| IBIS file stm32u3b5_3c5_lqfp100_smps.ibs
[IBIS ver] 4.2
[File name] stm32u3b5_3c5_lqfp100_smps.ibs
[File Rev] 0.1
[Date] 09-03-2026
[Source] Data Created at STMicroelectronics
[Notes]  File originated from ELDO simulations.
[Disclaimer]  This information is for modeling purpose only and is
   not guaranted. The information is subject to change without
   notice.
[Copyright] Copyright 2026 STMicroelectronics Inc.
|   Component stm32u3b5_3c5_lqfp100_smps
[Component] stm32u3b5_3c5_lqfp100_smps
[Manufacturer] STMicroelectronics
[Package]
| variable   typ   min   max
R_pkg  0  NA  NA
L_pkg  0  NA  NA
C_pkg  0  NA  NA
[Pin]   signal_name   model_name
1  PE2  io8_ft_100m
2  PE3  io8_ft_100m_hslv
3  PE4  io8_ft_100m
4  PE5  io8_ft_100m
5  PE6  io8_ft_100m
6  VBAT  power
7  PC13  io8_ft_100m_v33
8  PC14-OSC32_IN  io_ft_tamp
9  PC15-OSC32_OUT  io_ft_tamp
10  VSS  gnd
11  VDD  power
12  PH0-OSC_IN  io8_ft_100m
13  PH1-OSC_OUT  io8_ft_100m
14  NRST  ioreset_v33
15  PC0  io8_ft_100m_hslv
16  PC1  io8_ft_100m_hslv
17  PC2  io8_ft_100m_hslv
18  PC3  io8_ft_100m_hslv
19  VSSA_VREFM  nc
20  VREFP  nc
21  VDDA  nc
22  PA0  io8_ft_100m
23  PA1  io8_ft_100m_hslv
24  PA2  io8_ft_100m_hslv
25  PA3  io8_ft_100m_hslv
26  VSS  gnd
27  VDD  power
28  PA4  io8_ft_100m_hslv
29  PA5  io8_ft_100m
30  PA6  io8_ft_100m_hslv
31  PA7  io8_ft_100m_hslv
32  PB0  io8_ft_100m_hslv
33  PB1  io8_ft_100m_hslv
34  PB2  io8_ft_100m_hslv
35  PE7  io8_ft_100m
36  PE8  io8_ft_100m
37  PE9  io8_ft_100m_hslv
38  PE10  io8_ft_100m_hslv
39  PE11  io8_ft_100m_hslv
40  PE12  io8_ft_100m_hslv
41  PE13  io8_ft_100m_hslv
42  PE14  io8_ft_100m_hslv
43  PE15  io8_ft_100m_hslv
44  PB10  io8_ft_100m_hslv
45  PB11  io8_ft_100m_hslv
46  VLXSMPS  nc
47  VDDSMPS  nc
48  VSSSMPS  nc
49  VDD11  nc
50  VSS  gnd
51  VDD  power
52  PB13  io8_ft_100m_hslv
53  PB14  io8_ft_100m_hslv
54  PB15  io8_ft_100m
55  PD8  io8_ft_100m
56  PD9  io8_ft_100m
57  PD10  io8_ft_100m
58  PD11  io8_ft_100m_hslv
59  PD12  io8_ft_100m_hslv
60  PD13  io8_ft_100m_hslv
61  PD14  io8_ft_100m
62  PD15  io8_ft_100m
63  PC6  io8_ft_100m_hslv
64  PC7  io8_ft_100m_hslv
65  PC8  io8_ft_100m_hslv
66  PC9  io8_ft_100m_hslv
67  PA8  io8_ft_100m_hslv
68  PA9  io8_ft_100m
69  PA10  io8_ft_100m
70  PA11  io8usb_ft_phy
71  PA12  io8usb_ft_phy
72  PA13  io8_ft_100m
73  VDDUSB  power
74  VSS  gnd
75  VDD  power
76  PA14  io8_ft_100m
77  PA15  io8_ft_100m
78  PC10  io8_ft_100m_hslv
79  PC11  io8_ft_100m_hslv
80  PC12  io8_ft_100m_hslv
81  PD0  io8_ft_100m
82  PD1  io8_ft_100m
83  PD2  io8_ft_100m_hslv
84  PD3  io8_ft_100m_hslv
85  PD4  io8_ft_100m_hslv
86  PD5  io8_ft_100m_hslv
87  PD6  io8_ft_100m_hslv
88  PD7  io8_ft_100m_hslv
89  PB3  io8_ft_100m_hslv
90  PB4  io8_ft_100m_hslv
91  PB5  io8_ft_100m_hslv
92  PB6  io8_ft_100m_hslv
93  PB7  io8_ft_100m_hslv
94  PH3-BOOT0  io8_ft_100m_hslv
95  PB8  io8_ft_100m_hslv
96  PB9  io8_ft_100m_hslv
97  PE0  io8_ft_100m
98  VDD11  nc
99  VSS  gnd
100  VDD  power
[Package Model]   42a-lqfp-14x14-100-251212
[Pin Mapping]   pulldown_ref   pullup_ref   | Comment
1  gndio  vddio
2  gndio  vddio
3  gndio  vddio
4  gndio  vddio
5  gndio  vddio
6  nc  vsw
7  gndio  vsw
8  gndio  vsw
9  gndio  vsw
10  gndio  nc
11  nc  vddio
12  gndio  vddio
13  gndio  vddio
14  gndio  vddio
15  gndio  vddio
16  gndio  vddio
17  gndio  vddio
18  gndio  vddio
19  nc  nc
20  nc  nc
21  nc  nc
22  gndio  vddio
23  gndio  vddio
24  gndio  vddio
25  gndio  vddio
26  gndio  nc
27  nc  vddio
28  gndio  vddio
29  gndio  vddio
30  gndio  vddio
31  gndio  vddio
32  gndio  vddio
33  gndio  vddio
34  gndio  vddio
35  gndio  vddio
36  gndio  vddio
37  gndio  vddio
38  gndio  vddio
39  gndio  vddio
40  gndio  vddio
41  gndio  vddio
42  gndio  vddio
43  gndio  vddio
44  gndio  vddio
45  gndio  vddio
46  nc  nc
47  nc  nc
48  nc  nc
49  nc  nc
50  gndio  nc
51  nc  vddio
52  gndio  vddio
53  gndio  vddio
54  gndio  vddio
55  gndio  vddio
56  gndio  vddio
57  gndio  vddio
58  gndio  vddio
59  gndio  vddio
60  gndio  vddio
61  gndio  vddio
62  gndio  vddio
63  gndio  vddio
64  gndio  vddio
65  gndio  vddio
66  gndio  vddio
67  gndio  vddio
68  gndio  vddio
69  gndio  vddio
70  gndio  vddusb  | Depending on IO usage
| 70  gndio  vddio  | Depending on IO usage
71  gndio  vddusb  | Depending on IO usage
| 71  gndio  vddio  | Depending on IO usage
72  gndio  vddio
73  nc  vddusb
74  gndio  nc
75  nc  vddio
76  gndio  vddio
77  gndio  vddio
78  gndio  vddio
79  gndio  vddio
80  gndio  vddio
81  gndio  vddio
82  gndio  vddio
83  gndio  vddio
84  gndio  vddio
85  gndio  vddio
86  gndio  vddio
87  gndio  vddio
88  gndio  vddio
89  gndio  vddio
90  gndio  vddio
91  gndio  vddio
92  gndio  vddio
93  gndio  vddio
94  gndio  vddio
95  gndio  vddio
96  gndio  vddio
97  gndio  vddio
98  nc  nc
99  gndio  nc
100  nc  vddio
|[Diff Pin]  inv_pin  vdiff  tdelay_typ  tdelay_min  tdelay_max
|71  70  NA  NA  NA  NA
[Model Selector] io8_ft_100m
io8_ft_100m_ls_1v2  "GPIO 100MHz - 5V tolerant - low speed - 1.2V range"
io8_ft_100m_ls_1v8  "GPIO 100MHz - 5V tolerant - low speed - 1.8V range"
io8_ft_100m_ls_3v3  "GPIO 100MHz - 5V tolerant - low speed - 3.3V range"
io8_ft_100m_ms_1v2  "GPIO 100MHz - 5V tolerant - med speed - 1.2V range"
io8_ft_100m_ms_1v8  "GPIO 100MHz - 5V tolerant - med speed - 1.8V range"
io8_ft_100m_ms_3v3  "GPIO 100MHz - 5V tolerant - med speed - 3.3V range"
io8_ft_100m_fs_1v2  "GPIO 100MHz - 5V tolerant - fast speed - 1.2V range"
io8_ft_100m_fs_1v8  "GPIO 100MHz - 5V tolerant - fast speed - 1.8V range"
io8_ft_100m_fs_3v3  "GPIO 100MHz - 5V tolerant - fast speed - 3.3V range"
io8_ft_100m_hs_1v2  "GPIO 100MHz - 5V tolerant - high speed - 1.2V range"
io8_ft_100m_hs_1v8  "GPIO 100MHz - 5V tolerant - high speed - 1.8V range"
io8_ft_100m_hs_3v3  "GPIO 100MHz - 5V tolerant - high speed - 3.3V range"
[Model Selector] io8_ft_100m_hslv
io8_ft_100m_ls_1v2  "GPIO 100MHz - 5V tolerant - low speed - 1.2V range"
io8_ft_100m_ls_1v8  "GPIO 100MHz - 5V tolerant - low speed - 1.8V range"
io8_ft_100m_ls_3v3  "GPIO 100MHz - 5V tolerant - low speed - 3.3V range"
io8_ft_100m_ms_1v2  "GPIO 100MHz - 5V tolerant - med speed - 1.2V range"
io8_ft_100m_ms_1v8  "GPIO 100MHz - 5V tolerant - med speed - 1.8V range"
io8_ft_100m_ms_3v3  "GPIO 100MHz - 5V tolerant - med speed - 3.3V range"
io8_ft_100m_fs_1v2  "GPIO 100MHz - 5V tolerant - fast speed - 1.2V range"
io8_ft_100m_fs_1v8  "GPIO 100MHz - 5V tolerant - fast speed - 1.8V range"
io8_ft_100m_fs_3v3  "GPIO 100MHz - 5V tolerant - fast speed - 3.3V range"
io8_ft_100m_hs_1v2  "GPIO 100MHz - 5V tolerant - high speed - 1.2V range"
io8_ft_100m_hs_1v8  "GPIO 100MHz - 5V tolerant - high speed - 1.8V range"
io8_ft_100m_hs_3v3  "GPIO 100MHz - 5V tolerant - high speed - 3.3V range"
io8_ft_100m_hslv_ls_1v2  "GPIO 100MHz low voltage optimization - 5V tolerant - low speed - 1.2V range"
io8_ft_100m_hslv_ls_1v8  "GPIO 100MHz low voltage optimization - 5V tolerant - low speed - 1.8V range"
io8_ft_100m_hslv_ls_2v5  "GPIO 100MHz low voltage optimization - 5V tolerant - low speed - 3.3V range"
io8_ft_100m_hslv_ms_1v2  "GPIO 100MHz low voltage optimization - 5V tolerant - med speed - 1.2V range"
io8_ft_100m_hslv_ms_1v8  "GPIO 100MHz low voltage optimization - 5V tolerant - med speed - 1.8V range"
io8_ft_100m_hslv_ms_2v5  "GPIO 100MHz low voltage optimization - 5V tolerant - med speed - 3.3V range"
io8_ft_100m_hslv_fs_1v2  "GPIO 100MHz low voltage optimization - 5V tolerant - fast speed - 1.2V range"
io8_ft_100m_hslv_fs_1v8  "GPIO 100MHz low voltage optimization - 5V tolerant - fast speed - 1.8V range"
io8_ft_100m_hslv_fs_2v5  "GPIO 100MHz low voltage optimization - 5V tolerant - fast speed - 3.3V range"
io8_ft_100m_hslv_hs_1v2  "GPIO 100MHz low voltage optimization - 5V tolerant - high speed - 1.2V range"
io8_ft_100m_hslv_hs_1v8  "GPIO 100MHz low voltage optimization - 5V tolerant - high speed - 1.8V range"
io8_ft_100m_hslv_hs_2v5  "GPIO 100MHz low voltage optimization - 5V tolerant - high speed - 3.3V range"
[Model Selector] io8_ft_100m_v33
io8_ft_100m_v33_ls_1v2  "GPIO_V33 100MHz - 5V tolerant - low speed - 1.2V range"
io8_ft_100m_v33_ls_1v8  "GPIO_V33 100MHz - 5V tolerant - low speed - 1.8V range"
io8_ft_100m_v33_ls_3v3  "GPIO_V33 100MHz - 5V tolerant - low speed - 3.3V range"
io8_ft_100m_v33_ms_1v2  "GPIO_V33 100MHz - 5V tolerant - med speed - 1.2V range"
io8_ft_100m_v33_ms_1v8  "GPIO_V33 100MHz - 5V tolerant - med speed - 1.8V range"
io8_ft_100m_v33_ms_3v3  "GPIO_V33 100MHz - 5V tolerant - med speed - 3.3V range"
io8_ft_100m_v33_fs_1v2  "GPIO_V33 100MHz - 5V tolerant - fast speed - 1.2V range"
io8_ft_100m_v33_fs_1v8  "GPIO_V33 100MHz - 5V tolerant - fast speed - 1.8V range"
io8_ft_100m_v33_fs_3v3  "GPIO_V33 100MHz - 5V tolerant - fast speed - 3.3V range"
io8_ft_100m_v33_hs_1v2  "GPIO_V33 100MHz - 5V tolerant - high speed - 1.2V range"
io8_ft_100m_v33_hs_1v8  "GPIO_V33 100MHz - 5V tolerant - high speed - 1.8V range"
io8_ft_100m_v33_hs_3v3  "GPIO_V33 100MHz - 5V tolerant - high speed - 3.3V range"
[Model Selector] io8usb_ft_phy
io8_ft_100m_ls_1v2  "GPIO 100MHz - 5V tolerant - low speed - 1.2V range"
io8_ft_100m_ls_1v8  "GPIO 100MHz - 5V tolerant - low speed - 1.8V range"
io8_ft_100m_ls_3v3  "GPIO 100MHz - 5V tolerant - low speed - 3.3V range"
io8_ft_100m_ms_1v2  "GPIO 100MHz - 5V tolerant - med speed - 1.2V range"
io8_ft_100m_ms_1v8  "GPIO 100MHz - 5V tolerant - med speed - 1.8V range"
io8_ft_100m_ms_3v3  "GPIO 100MHz - 5V tolerant - med speed - 3.3V range"
io8_ft_100m_fs_1v2  "GPIO 100MHz - 5V tolerant - fast speed - 1.2V range"
io8_ft_100m_fs_1v8  "GPIO 100MHz - 5V tolerant - fast speed - 1.8V range"
io8_ft_100m_fs_3v3  "GPIO 100MHz - 5V tolerant - fast speed - 3.3V range"
io8_ft_100m_hs_1v2  "GPIO 100MHz - 5V tolerant - high speed - 1.2V range"
io8_ft_100m_hs_1v8  "GPIO 100MHz - 5V tolerant - high speed - 1.8V range"
io8_ft_100m_hs_3v3  "GPIO 100MHz - 5V tolerant - high speed - 3.3V range"
io8usb_ft_phy_hs_3v3   "USB full speed"
io8usb_ft_phy_ls_3v3   "USB low speed"
[Model Selector] io_ft_tamp
io_ft_tamp_ls_1v2 "io8_ft tamp low speed @ 1.2V"
io_ft_tamp_ls_1v8 "io8_ft tamp low speed @ 1.8V"
io_ft_tamp_ls_3v3 "io8_ft tamp low speed @ 3.3V"
io_ft_tamp_ms_1v2 "io8_ft tamp med speed @ 1.2V"
io_ft_tamp_ms_1v8 "io8_ft tamp med speed @ 1.8V"
io_ft_tamp_ms_3v3 "io8_ft tamp med speed @ 3.3V"
io_ft_tamp_fs_1v2 "io8_ft tamp fast speed @ 1.2V"
io_ft_tamp_fs_1v8 "io8_ft tamp fast speed @ 1.8V"
io_ft_tamp_fs_3v3 "io8_ft tamp fast speed @ 3.3V"
io_ft_tamp_hs_1v2 "io8_ft tamp high speed @ 1.2V"
io_ft_tamp_hs_1v8 "io8_ft tamp high speed @ 1.8V"
io_ft_tamp_hs_3v3 "io8_ft tamp high speed @ 3.3V"
[Model Selector] ioreset_v33
ioreset_v33_1v2 "Reset PAD. 5V tolerant. 1.2V range"
ioreset_v33_1v8 "Reset PAD. 5V tolerant. 1.8V range"
ioreset_v33_3v3 "Reset PAD. 5V tolerant. 3.3V range"
[Define Package Model]  42a-lqfp-14x14-100-251212
[Manufacturer]  Unknown
[OEM]  Unknown
[Description]  None
[Number Of Pins]  96
[Pin Numbers]
| Pin Num   Terminal Name
14 | NRST
22 | PA0
23 | PA1
24 | PA2
25 | PA3
28 | PA4
29 | PA5
30 | PA6
31 | PA7
67 | PA8
68 | PA9
69 | PA10
70 | PA11
71 | PA12
72 | PA13
76 | PA14
77 | PA15
32 | PB0
33 | PB1
34 | PB2
89 | PB3
90 | PB4
91 | PB5
92 | PB6
93 | PB7
95 | PB8
96 | PB9
44 | PB10
45 | PB11
52 | PB13
53 | PB14
54 | PB15
15 | PC0
16 | PC1
17 | PC2
18 | PC3
63 | PC6
64 | PC7
65 | PC8
66 | PC9
78 | PC10
79 | PC11
80 | PC12
7 | PC13
8 | PC14-OSC32_IN
9 | PC15-OSC32_OUT
81 | PD0
82 | PD1
83 | PD2
84 | PD3
85 | PD4
86 | PD5
87 | PD6
88 | PD7
55 | PD8
56 | PD9
57 | PD10
58 | PD11
59 | PD12
60 | PD13
61 | PD14
62 | PD15
97 | PE0
1 | PE2
2 | PE3
3 | PE4
4 | PE5
5 | PE6
35 | PE7
36 | PE8
37 | PE9
38 | PE10
39 | PE11
40 | PE12
41 | PE13
42 | PE14
43 | PE15
12 | PH0-OSC_IN
13 | PH1-OSC_OUT
94 | PH3-BOOT0
49 | VDD11
98 | VDD11
6 | VBAT
11 | VDD
27 | VDD
51 | VDD
75 | VDD
100 | VDD
21 | VDDA
47 | VDDSMPS
73 | VDDUSB
46 | VLXSMPS
20 | VREFP
10 | VSS
19 | VSSA_VREFM
48 | VSSSMPS
|[Merged Pins]  10
|26  |  VSS
|50  |  VSS
|74  |  VSS
|99  |  VSS
[Model Data]
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[End Model Data]
[End Package Model]
|End [Component]
| Models and submodels in the file (53): io8_ft_100m_fs_1v2 (I/O), io8_ft_100m_fs_1v8 (I/O), io8_ft_100m_fs_3v3 (I/O), io8_ft_100m_hs_1v2 (I/O), io8_ft_100m_hs_1v8 (I/O), io8_ft_100m_hs_3v3 (I/O), io8_ft_100m_hslv_fs_1v2 (I/O), io8_ft_100m_hslv_fs_1v8 (I/O), io8_ft_100m_hslv_fs_2v5 (I/O), io8_ft_100m_hslv_hs_1v2 (I/O), io8_ft_100m_hslv_hs_1v8 (I/O), io8_ft_100m_hslv_hs_2v5 (I/O), io8_ft_100m_hslv_ls_1v2 (I/O), io8_ft_100m_hslv_ls_1v8 (I/O), io8_ft_100m_hslv_ls_2v5 (I/O), io8_ft_100m_hslv_ms_1v2 (I/O), io8_ft_100m_hslv_ms_1v8 (I/O), io8_ft_100m_hslv_ms_2v5 (I/O), io8_ft_100m_ls_1v2 (I/O), io8_ft_100m_ls_1v8 (I/O), io8_ft_100m_ls_3v3 (I/O), io8_ft_100m_ms_1v2 (I/O), io8_ft_100m_ms_1v8 (I/O), io8_ft_100m_ms_3v3 (I/O), io8_ft_100m_v33_fs_1v2 (I/O), io8_ft_100m_v33_fs_1v8 (I/O), io8_ft_100m_v33_fs_3v3 (I/O), io8_ft_100m_v33_hs_1v2 (I/O), io8_ft_100m_v33_hs_1v8 (I/O), io8_ft_100m_v33_hs_3v3 (I/O), io8_ft_100m_v33_ls_1v2 (I/O), io8_ft_100m_v33_ls_1v8 (I/O), io8_ft_100m_v33_ls_3v3 (I/O), io8_ft_100m_v33_ms_1v2 (I/O), io8_ft_100m_v33_ms_1v8 (I/O), io8_ft_100m_v33_ms_3v3 (I/O), io8usb_ft_phy_hs_3v3 (I/O), io8usb_ft_phy_ls_3v3 (I/O), io_ft_tamp_fs_1v2 (I/O), io_ft_tamp_fs_1v8 (I/O), io_ft_tamp_fs_3v3 (I/O), io_ft_tamp_hs_1v2 (I/O), io_ft_tamp_hs_1v8 (I/O), io_ft_tamp_hs_3v3 (I/O), io_ft_tamp_ls_1v2 (I/O), io_ft_tamp_ls_1v8 (I/O), io_ft_tamp_ls_3v3 (I/O), io_ft_tamp_ms_1v2 (I/O), io_ft_tamp_ms_1v8 (I/O), io_ft_tamp_ms_3v3 (I/O), ioreset_v33_1v2 (I/O_open_drain), ioreset_v33_1v8 (I/O_open_drain), ioreset_v33_3v3 (I/O_open_drain)
